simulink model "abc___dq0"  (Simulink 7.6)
settings: Solver=FixedStepDiscrete  SolverMode=SingleTasking  StartTime=0.0  StopTime=0.15  MaxStep=200e-6  RelTol=1e-3  AbsTol=1e-2
libraries: powerlib_extras x5

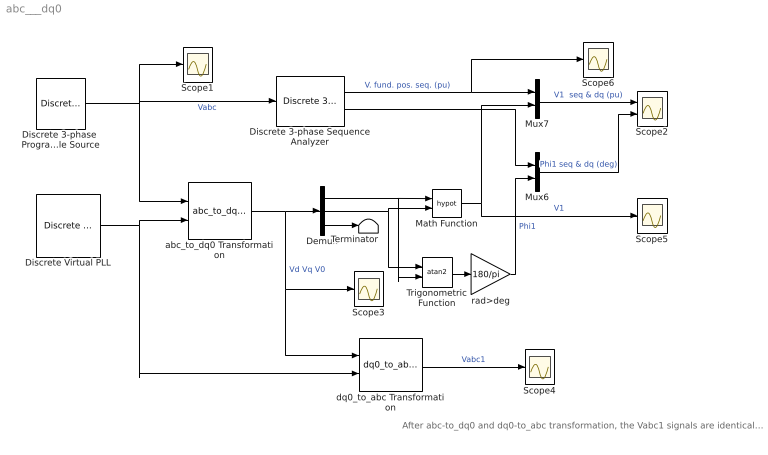
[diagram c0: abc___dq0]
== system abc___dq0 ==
  note: After abc-to_dq0 and dq0-to_abc transformation, the Vabc1 signals are identical to the original Vabc signals
  Demux : Demux  Outputs=3
  Discrete 3-phase  Programmable Source : powerlib_extras/Discrete  Control Blocks/Discrete 3-phase  Programmable Source  DialogController=POWERSYS.PowerSysDialog  SystemSampleTime=-1  Par_Vps="[1.0  15  60]"  VariationEntity=Amplitude  VariationType=Step  VariationStep=0.5  VariationRate=10  VariationMag=0.3  VariationFreq=2  Par_Timing_Variation=[0.05 1]  SinglePhase=on  Yampli=[1 0.2 1.2 1.0]  Xtime=[0 0.1 0.15 0.2]  HarmonicGeneration=off  Par_HarmoA=[1 0.3 -30 2]  Par_HarmoB=[1 0.0 0.0 1]  Par_Timing_Harmo="[0.1  1]"  Ts=50e-6
  Discrete Virtual PLL : powerlib_extras/Discrete  Control Blocks/Discrete Virtual PLL  DialogController=POWERSYS.PowerSysDialog  SystemSampleTime=-1  Freq=60  Phase=0  Ts=50e-6
  Discrete 3-phase Sequence Analyzer : powerlib_extras/Discrete Measurements/Discrete 3-phase Sequence Analyzer  DialogController=POWERSYS.PowerSysDialog  SystemSampleTime=-1  Freq=60  n=1  seq=Positive  Par_Init=[1 15]  Ts=50e-6
  Math Function : Math  Operator=hypot
  Mux6 : Mux  Inputs=2
  Mux7 : Mux  Inputs=2
  Scope{1,3..6} (5 alike) : Scope
  Scope2 : Scope  NumInputPorts=2
  Terminator : Terminator
  Trigonometric Function : Trigonometry  Operator=atan2
  abc_to_dq0 Transformation : powerlib_extras/Measurements/abc_to_dq0 Transformation  DialogController=POWERSYS.PowerSysDialog  SystemSampleTime=-1
  dq0_to_abc Transformation : powerlib_extras/Measurements/dq0_to_abc Transformation  DialogController=POWERSYS.PowerSysDialog  SystemSampleTime=-1
  rad>deg : Gain  Gain=180/pi
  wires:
  Demux/2 -> Math Function/2, Trigonometric Function/1
  Demux/1 -> Math Function/1, Trigonometric Function/2
  Math Function/1 -> Mux7/2, Scope5/1  "V1"
  Discrete 3-phase Sequence Analyzer/1 -> Mux7/1, Scope6/1  "V. fund. pos. seq. (pu)"
  Discrete 3-phase Sequence Analyzer/2 -> Mux6/1
  abc_to_dq0 Transformation/1 -> Demux/1, Scope3/1, dq0_to_abc Transformation/1  "Vd Vq V0"
  Trigonometric Function/1 -> rad>deg/1
  rad>deg/1 -> Mux6/2  "Phi1"
  dq0_to_abc Transformation/1 -> Scope4/1  "Vabc1"
  Mux6/1 -> Scope2/2  "Phi1 seq & dq (deg)"
  Mux7/1 -> Scope2/1  "V1  seq & dq (pu)"
  Discrete 3-phase  Programmable Source/1 -> Scope1/1, Discrete 3-phase Sequence Analyzer/1, abc_to_dq0 Transformation/1  "Vabc"
  Discrete Virtual PLL/2 -> abc_to_dq0 Transformation/2, dq0_to_abc Transformation/2
  Demux/3 -> Terminator/1
